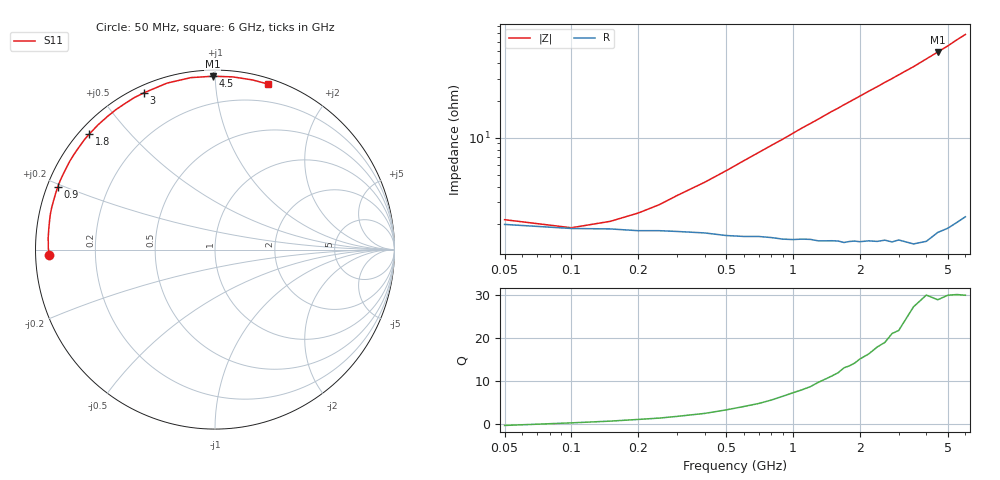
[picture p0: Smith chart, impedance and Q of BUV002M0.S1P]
! Infineon Technologies  Discrete & RF Semiconductors
! BB 833
! Si Tuning Diode in SOD323
! VR =
! S-Parameters:  June  1999
# GHz  S  MA  R  50
!  f  S11
! GHz  MAG  ANG
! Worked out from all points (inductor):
!   34 points, 50 MHz to 6 GHz, reference 50 ohm
!   read as one part to ground: L = 1.69 nH near 500 MHz
!   highest Q = 30 at 4.5 GHz (marker M1), where L = 1.75 nH
!   S11 on the Smith chart (normalised r, x): 50 MHz: 0.04, -0.02; 900 MHz: 0.03, +0.19; 1.8 GHz: 0.03, +0.39; 3 GHz: 0.03, +0.65; 4.5 GHz: 0.03, +0.99; 6 GHz: 0.05, +1.37
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0.05  0.9236 -178.0
0.1  0.929 179.3
0.2  0.9318 176.1
0.25  0.9319 174.8
0.3  0.9329 173.3
0.5  0.9381 168.2
0.6  0.9395 165.6
0.8  0.9414 160.6
0.9  0.9434 158.2
1.1  0.9445 153.2
1.2  0.9453 150.9
1.3  0.9472 148.6
1.4  0.9478 146.2
1.6  0.9493 141.8
1.7  0.9513 139.5
1.8  0.9511 137.4
2  0.9527 133.2
2.2  0.9534 129.1
2.4  0.9554 125.3
2.6  0.956 121.4
2.8  0.9588 117.9
3  0.9589 114.3
3.5  0.9654 106.1
4  0.9675 98.0
4.5  0.966 90.7
5  0.9674 84.1
5.5  0.9681 77.6
6  0.9687 72.2
